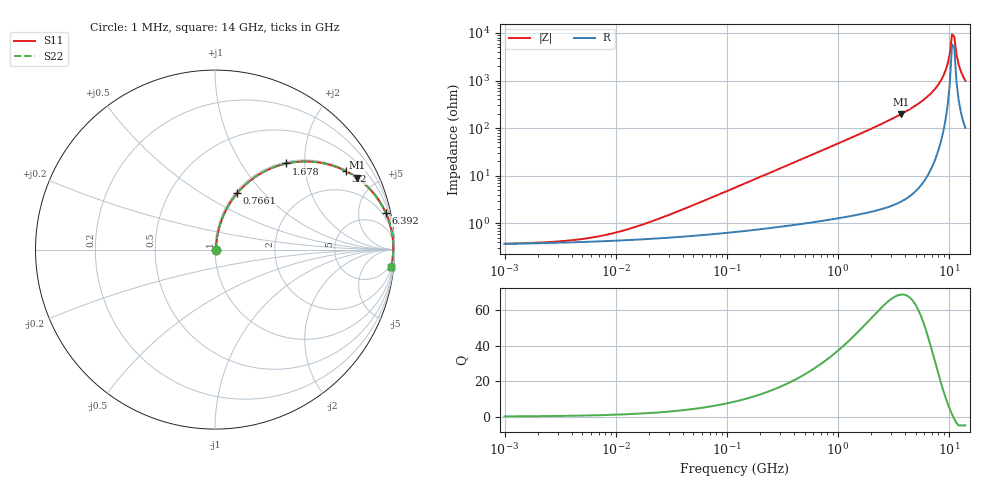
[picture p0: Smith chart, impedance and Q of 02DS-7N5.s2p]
# MHz S MA R 50
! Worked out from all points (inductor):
!   208 points, 1 MHz to 14 GHz, reference 50 ohm
!   read as one part in series: L = 7.5 nH near 33.29 MHz
!   highest Q = 68.8 at 3.675 GHz (marker M1), where L = 8.47 nH
!   self-resonance near 10.62 GHz
!   S11 on the Smith chart (normalised r, x): 1 MHz: 1.01, +0.00; 766.1 MHz: 1.02, +0.73; 1.678 GHz: 1.03, +1.62; 3.2 GHz: 1.05, +3.30; 6.392 GHz: 1.20, +9.23; 14 GHz: 3, -20
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1  0.003706 7.3  0.9963 -0.0  0.9963 -0.0  0.003706 7.3
5.02384  0.004672 30.2  0.996 -0.1  0.996 -0.1  0.004672 30.2
11.0037  0.006747 49.6  0.9956 -0.3  0.9956 -0.3  0.006747 49.6
25.239  0.01278 67.1  0.9951 -0.7  0.9951 -0.7  0.01278 67.1
121.082  0.05698 80.2  0.9919 -3.2  0.9919 -3.2  0.05698 80.2
277.723  0.1291 79.0  0.9836 -7.4  0.9836 -7.4  0.1291 79.0
580.879  0.2624 72.6  0.9551 -15.2  0.9551 -15.2  0.2624 72.6
766.06  0.3378 68.5  0.9306 -19.7  0.9306 -19.7  0.3378 68.5
1677.9  0.6236 50.3  0.7696 -38.6  0.7696 -38.6  0.6236 50.3
2918.24  0.8233 33.7  0.5553 -55.4  0.5553 -55.4  0.8233 33.7
3200.23  0.8499 31.0  0.5145 -58.2  0.5145 -58.2  0.8499 31.0
3675.1  0.8853 26.9  0.4524 -62.3  0.4524 -62.3  0.8853 26.9
6391.82  0.973 12.2  0.2108 -76.6  0.2108 -76.6  0.973 12.2
8049.57  0.9882 6.7  0.1171 -80.9  0.1171 -80.9  0.9882 6.7
9244.04  0.9924 3.6  0.06257 -81.3  0.06257 -81.3  0.9924 3.6
9680.35  0.9931 2.5  0.04467 -79.9  0.04467 -79.9  0.9931 2.5
10137.3  0.9934 1.5  0.02704 -75.1  0.02704 -75.1  0.9934 1.5
10615.7  0.9933 0.5  0.01069 -51.0  0.01069 -51.0  0.9933 0.5
11116.8  0.9929 -0.5  0.01188 52.8  0.01188 52.8  0.9929 -0.5
11641.5  0.992 -1.6  0.02846 72.9  0.02846 72.9  0.992 -1.6
12191  0.9908 -2.6  0.04606 77.2  0.04606 77.2  0.9908 -2.6
14000  0.9848 -5.7  0.09976 78.4  0.09976 78.4  0.9848 -5.7
